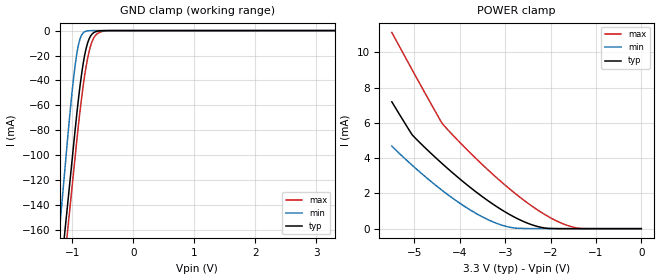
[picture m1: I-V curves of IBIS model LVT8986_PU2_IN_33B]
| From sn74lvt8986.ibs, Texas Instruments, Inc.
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[Model]   LVT8986_PU2_IN_33B
Model_type  Input
Vinl=0.8
Vinh=2.0
| variable   typ   min   max
C_comp   3.18pF   2.51pF   4.48pF
[Temperature Range]   40   -40   100
| Ambient temperature   25   -40   85
[Voltage range]   3.3   2.7   3.6
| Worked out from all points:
|   GND clamp passes 1 mA (typ) near -0.62 V on its own axis
|   POWER clamp passes 1 mA (typ) near -3.03 V on its own axis
[GND Clamp]
| LVT8986_PU2_IN_33B
|   Voltage   I(typ)   I(min)   I(max)
-5.5V     -2.287A    -2.545A    -2.286A
-1.23V    -213.2mA   -170.8mA   -233.6mA
-1.2V     -198.6mA   -154.2mA   -219.2mA
-1.13V    -164.7mA   -115.4mA   -185.6mA
-1.105V   -152.6mA   -101.6mA   -173.6mA
-1.075V   -138.1mA   -85mA      -159.2mA
-975mV    -89.69mA   -36mA      -111.2mA
-900mV    -54.93mA   -11.38mA   -75.88mA
-775mV    -14.5mA    -474.9uA   -29.04mA
-700mV    -4.254mA   -33.37uA   -12.08mA
-600mV    -616.1uA   -10.07uA   -2.838mA
3.3V      16.16pA    8.699pA    -7.502nA
[POWER Clamp]
| LVT8986_PU2_IN_33B
|   Voltage   I(typ)   I(min)   I(max)
-5.5V     7.191mA    4.679mA    11.13mA
-5.055V   5.335mA    3.603mA    9.023mA
-4.39V    3.688mA    2.171mA    5.968mA
-3.895V   2.595mA    1.261mA    4.615mA
-3.45V    1.713mA    598.2uA    3.501mA
-3.055V   1.033mA    183.2uA    2.585mA
-2.715V   547.5uA    22.73uA    1.862mA
-2.17V    55.3uA     4.611nA    869.2uA
-1.83V    1.773uA    15.23pA    391.7uA
-1.525V   8.75nA     13.18pA    99.72uA
-1.26V    93.03pA    11.89pA    5.075uA
-95.1fV   16.16pA    5.854pA    469.5pA
